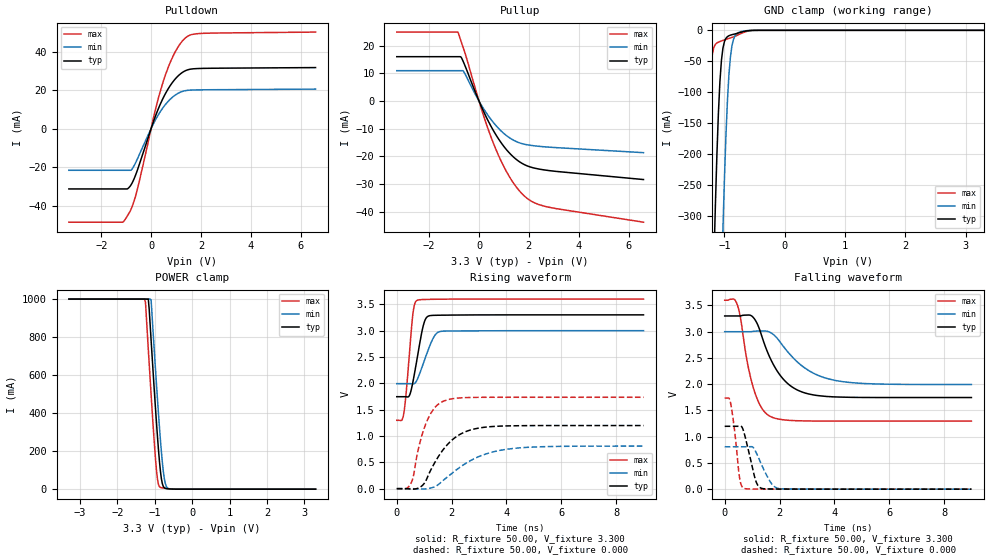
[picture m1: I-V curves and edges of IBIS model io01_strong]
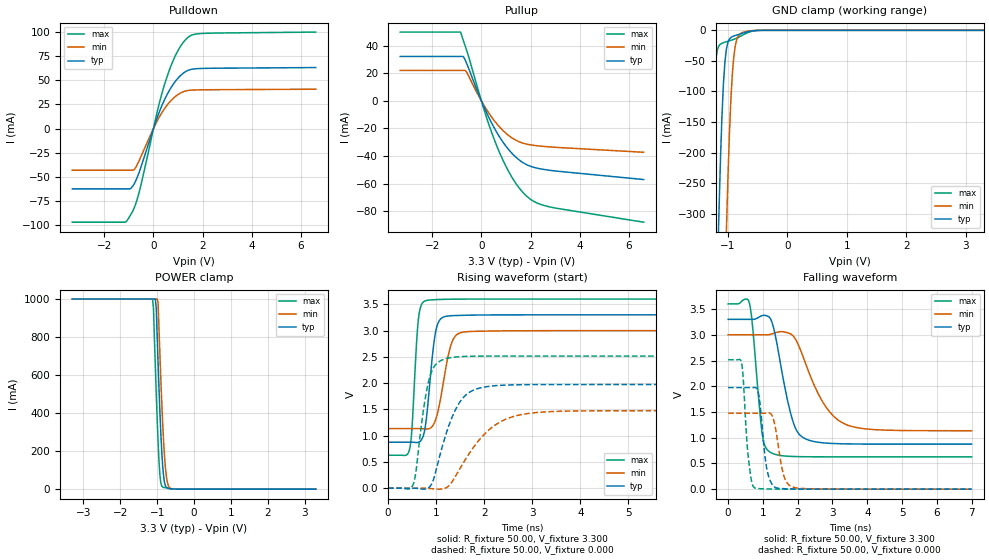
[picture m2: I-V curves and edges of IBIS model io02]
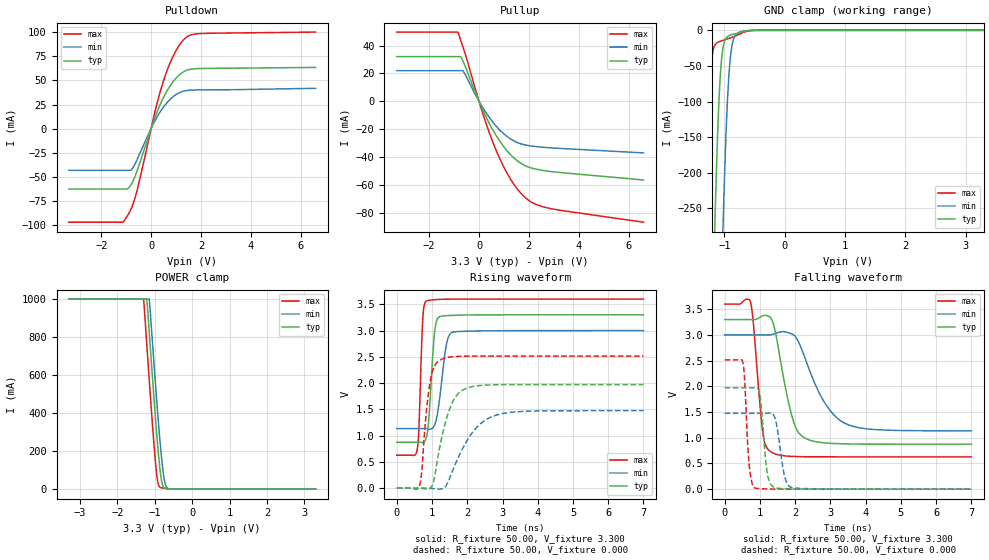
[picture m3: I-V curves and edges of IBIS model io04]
[IBIS Ver]   3.2
[File name]   rx63n_176lqfp.ibs
[File Rev]   1.00
[Date]   May 21, 2013
[Source]   From silicon level SPICE model at
   Renesas Electronics Corporation
[Notes]
|   Renesas Microcomputer RX631/RX63N Group
|   RX631/RX63N 176pin LQFP
|   VCCQ : 3.30V
|(1) This IBIS file checked the format with ibischk5.
|   Format Error and Warning are 0.
|(2) Temperature described Tj.
|   Tj[deg]
|   Typical   45.0
|   Minimum   105.0
|   Maximum   -40.0
|(3) History
|   Rev 0.50  2012.09.10
|   New creation by Renesas Electronics Corporation
|   Rev 1.00  2013.05.21
|   Only change of revision number.
|   by Renesas Electronics Corporation
[Disclaimer]
   This information is for modeling purposes only,
   and is not guaranteed.
[Copyright]   Copyright 2012, Renesas Electronics Corporation ,
   All Rights Reserved
[Component]   rx63n_176lqfp
[Manufacturer]  Renesas Electronics Corporation
[Package]
|   typ   min   max
R_pkg   254m   226m   289m
L_pkg   4.5nH   3.8nH   5.1nH
C_pkg   1.0pF   0.8pF   1.2pF
[Pin] signal_name   model_name
1   AVSS0   GND
2   P05   io02
3   VREFH   POWER
4   P03   io02
5   VREFL   GND
6   P02   io01
7   P01   io01
8   P00   io01
9   PF5   io04
10   EMLE   input06
11   PJ5   io04
12   VSS   GND
13   PJ3   io04
14   VCL   POWER
15   VBATT   POWER
16   NC   NC
17   PF4   io04
18   MD   io04
19   XCIN   NC
20   XCOUT   NC
21   RES#   input02
22   P37   io05
23   VSS   GND
24   P36   io03
25   VCC   POWER
26   P35   input01
27   P34   io04
28   P33   io06
29   P32   io21
30   PF3   io04
31   PF2   io04
32   P31   io21
33   P30   io21
34   PF1   io04
35   PF0   io04
36   P27   io07
37   P26   io07
38   P25   io04
39   VCC   POWER
40   P24   io04
41   VSS   GND
42   P23   io04
43   P22   io04
44   P21   io16
45   P20   io16
46   P17   io15
47   P87   io04
48   P16   io15
49   P86   io04
50   P15   io06
51   P14   io06
52   P85   io04
53   P13   io18
54   P12   io18
55   P11   io04
56   P10   io04
57   VCC_USB   POWER
58   USB0_DM   io09
59   USB0_DP   io09
60   VSS_USB   GND
61   P57   io07
62   P56   io07
63   USB1_DM   io09
64   USB1_DP   io09
65   VCC_USB   POWER
66   P55   io07
67   P54   io07
68   P53   io04
69   P84   io04
70   P52   io07
71   P51   io07
72   P50   io07
73   VSS   GND
74   P83   io04
75   VCC   POWER
76   PC7   io07
77   PC6   io07
78   PC5   io07
79   P82   io04
80   P81   io04
81   P80   io04
82   PC4   io07
83   PC3   io08
84   P77   io04
85   P76   io04
86   PC2   io08
87   P75   io04
88   P74   io04
89   PC1   io17
90   VCC   POWER
91   PC0   io17
92   VSS   GND
93   P73   io04
94   PB7   io07
95   PB6   io07
96   PB5   io07
97   PB4   io07
98   PB3   io07
99   PB2   io07
100   PB1   io07
101   P72   io04
102   P71   io04
103   VCC   POWER
104   PB0   io07
105   VSS   GND
106   PA7   io07
107   PA6   io07
108   PA5   io07
109   PA4   io07
110   PA3   io07
111   PG7   io07
112   PA2   io07
113   PG6   io07
114   PA1   io07
115   VCC   POWER
116   PG5   io04
117   VSS   GND
118   PA0   io07
119   PG4   io07
120   P67   io06
121   PG3   io07
122   P66   io04
123   PG2   io07
124   P65   io04
125   PE7   io01
126   PE6   io01
127   VCC   POWER
128   P70   io04
129   VSS   GND
130   PE5   io01
131   PE4   io01
132   PE3   io01
133   PE2   io01
134   PE1   io01
135   PE0   io01
136   P64   io04
137   P63   io04
138   P62   io04
139   P61   io04
140   VSS   GND
141   P60   io04
142   VCC   POWER
143   PD7   io01
144   PG1   io07
145   PD6   io01
146   PG0   io07
147   PD5   io01
148   PD4   io01
149   P97   io07
150   PD3   io01
151   VSS   GND
152   P96   io07
153   VCC   POWER
154   PD2   io01
155   P95   io07
156   PD1   io01
157   P94   io07
158   PD0   io01
159   P93   io01
160   P92   io01
161   P91   io01
162   VSS   GND
163   P90   io01
164   VCC   POWER
165   P47   io14
166   P46   io14
167   P45   io14
168   P44   io14
169   P43   io14
170   P42   io14
171   P41   io14
172   VREFL0   GND
173   P40   io14
174   VREFH0   POWER
175   AVCC0   POWER
176   P07   io06
[Diff Pin]   inv_pin   vdiff   tdelay_typ   tdelay_min   tdelay_max
58   59   0.000V   0.000s   NA   NA
63   64   0.000V   0.000s   NA   NA
[Model Selector]   io01
io01_strong   driver strength strong
io01_weak   driver strength weak
[Model Selector]   io07
io07_strong   driver strength strong
io07_weak   driver strength weak
[Model Selector]   io08
io08_strong   driver strength strong
io08_weak   driver strength weak
[Model Selector]   io15
io15a   driver strength strong
io15b   I2C buffer 1
[Model Selector]   io16
io16a   driver strength strong
io16b   I2C buffer 2
[Model Selector]   io17
io17a_strong   driver strength strong
io17a_weak   driver strength weak
io17b   I2C buffer 3
[Model Selector]   io18
io18a   driver strength strong
io18b   I2C buffer 4
| Models and submodels in the file (26): io01_strong (I/O), io01_weak (I/O), io02 (I/O), io03 (I/O), io04 (I/O), io05 (I/O), io06 (I/O), io07_strong (I/O), io07_weak (I/O), io08_strong (I/O), io08_weak (I/O), io09 (I/O), io14 (I/O), io15a (I/O), io15b (I/O_open_drain), io16a (I/O), io16b (I/O_open_drain), io17a_strong (I/O), io17a_weak (I/O), io17b (I/O_open_drain), io18a (I/O), io18b (I/O_open_drain), io21 (I/O), input01 (Input), input02 (Input), input06 (Input)
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[Model]   io01_strong
Model_type   I/O
Polarity   Non-Inverting
Enable   Active-High
Vinl  =   0.660V
Vinh  =   2.640V
Vmeas =   1.650V
Cref  =   30.00pF
| variable   typ   min   max
C_comp   5.910pF   5.910pF   5.910pF
| variable   typ   min   max
[Temperature Range]   45.000   105.000   -40.000
| variable   typ   min   max
[Voltage Range]   3.300V   3.000V   3.600V
| variable   typ   min   max
[Pullup Reference]   3.300V   3.000V   3.600V
| variable   typ   min   max
[Pulldown Reference]   0.000V   0.000V   0.000V
| variable   typ   min   max
[POWER Clamp Reference] 3.300V   3.000V   3.600V
| variable   typ   min   max
[GND Clamp Reference]   0.000V   0.000V   0.000V
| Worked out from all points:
|   slope of the pulldown table from 0 to 0.495 V, typ, clamps not added: 30.7 ohm
|   slope of the pullup table from 0 to 0.495 V, typ, clamps not added: 52.9 ohm
|   GND clamp passes 1 mA (typ) near -0.63 V on its own axis
|   POWER clamp passes 1 mA (typ) near -0.58 V on its own axis
|   rising waveform, R_fixture 50.00, V_fixture 3.300: 20-80 % time 321ps typ, 432ps min, 222ps max; typ from 1.75 V to 3.3 V
|   rising waveform, R_fixture 50.00, V_fixture 0.000: 20-80 % time 961ps typ, 1.48ns min, 553ps max; typ from 0 V to 1.2 V
|   falling waveform, R_fixture 50.00, V_fixture 3.300: 20-80 % time 902ps typ, 1.27ns min, 542ps max; typ from 3.3 V to 1.75 V
|   falling waveform, R_fixture 50.00, V_fixture 0.000: 20-80 % time 324ps typ, 446ps min, 218ps max; typ from 1.2 V to 0 V
[Pulldown]
| io01_strong Pulldown rx631_rx63n
| Thu Mar 22 17:15:49 2012
| voltage   I(typ)   I(min)   I(max)
-3.3V     -31.31mA   -21.63mA   -48.57mA
-1.15V    -31.31mA   -21.63mA   -48.57mA
-1.025V   -31.31mA   -21.63mA   -46.81mA
-800mV    -29.1mA    -21.49mA   -41.71mA
-600mV    -23.34mA   -17.13mA   -33.95mA
175mV     6.49mA     4.538mA    9.911mA
525mV     16.92mA    11.68mA    25.93mA
950mV     25.49mA    17.23mA    39.38mA
1.4V      30.18mA    19.75mA    47.31mA
1.7V      31.04mA    20.05mA    49.02mA
2.1V      31.26mA    20.14mA    49.45mA
6.6V      31.67mA    20.5mA     50.09mA
[Pullup]
| io01_strong Pullup rx631_rx63n
| Thu Mar 22 17:15:49 2012
| voltage   I(typ)   I(min)   I(max)
-3.3V     16.04mA    10.98mA    24.94mA
-850mV    16.04mA    10.98mA    24.94mA
-725mV    15.94mA    10.98mA    21.66mA
-625mV    14.1mA     10.75mA    19.05mA
175mV     -3.59mA    -2.649mA   -5.083mA
700mV     -12.53mA   -9.072mA   -17.96mA
1V        -16.45mA   -11.75mA   -23.79mA
1.325V    -19.76mA   -13.87mA   -28.89mA
1.95V     -23.51mA   -15.85mA   -35.33mA
2.3V      -24.41mA   -16.28mA   -37.1mA
2.9V      -25.25mA   -16.74mA   -38.59mA
6.6V      -28.4mA    -18.67mA   -43.82mA
[GND Clamp]
| io01_strong GNDClamp rx631_rx63n
| Thu Mar 22 17:15:49 2012
| voltage   I(typ)   I(min)   I(max)
-3.3V     -1A        -1A        -1A
-1.325V   -1A        -1A        -369.2mA
-1.3V     -928.6mA   -1A        -269.7mA
-1.25V    -694.8mA   -1A        -112.6mA
-1.175V   -376mA     -953.3mA   -27.44mA
-1.15V    -283.8mA   -837.7mA   -22.69mA
-1.075V   -83.42mA   -512.2mA   -18.16mA
-1.025V   -28.94mA   -323mA     -16.39mA
-925mV    -8.707mA   -71.38mA   -13.1mA
-850mV    -6.468mA   -14.65mA   -10.64mA
-675mV    -1.81mA    -1.082mA   -3.186mA
3.3V      0A         0A         0A
[POWER Clamp]
| io01_strong PWRClamp rx631_rx63n
| Thu Mar 22 17:15:49 2012
| voltage   I(typ)   I(min)   I(max)
-3.3V     1A         1A         1A
-1.275V   1A         1A         1A
-1.25V    1A         1A         982.1mA
-1.175V   1A         1A         736.6mA
-1.1V     784.3mA    995.9mA    498mA
-1V       476.2mA    683.1mA    204.7mA
-950mV    332.1mA    533mA      87.52mA
-875mV    143.3mA    321.7mA    12.76mA
-825mV    55.42mA    197.2mA    7.873mA
-750mV    8.12mA     59.94mA    5.513mA
-625mV    1.619mA    2.607mA    2.132mA
3.3V      0A         0A         0A
[Ramp]
dV/dt_r   0.719/960.74p  0.485/1.48n   1.041/552.35p
dV/dt_f   0.933/901.13p  0.604/1.27n   1.382/541.71p
R_load = 50.00ohm
[Rising Waveform]
| io01_strong Rising-High rx631_rx63n
| Thu Mar 22 17:15:49 2012
R_fixture = 50.00
V_fixture = 3.300
V_fixture_min = 3.000
V_fixture_max = 3.600
C_fixture = 0.00pF
| Time   V(typ)   V(min)   V(max)
0s        1.746V     1.994V     1.297V
250ps     1.746V     1.994V     1.413V
450ps     1.759V     1.994V     2.489V
580ps     2.004V     1.989V     3.28V
645ps     2.183V     1.996V     3.491V
740ps     2.465V     2.064V     3.575V
1.045ns   3.216V     2.49V      3.592V
1.35ns    3.291V     2.878V     3.596V
1.585ns   3.293V     2.985V     3.598V
9ns       3.3V       3V         3.6V
[Rising Waveform]
| io01_strong Rising-Low rx631_rx63n
| Thu Mar 22 17:15:49 2012
R_fixture = 50.00
V_fixture = 0.000
C_fixture = 0.00pF
| Time   V(typ)   V(min)   V(max)
0s        0V         0V         0V
510ps     -7mV       0V         95mV
605ps     -9mV       -1mV       236mV
840ps     25mV       -7mV       868mV
1.075ns   164mV      -4mV       1.25V
1.385ns   494mV      37mV       1.537V
1.755ns   781mV      183mV      1.672V
2.55ns    1.09V      490mV      1.729V
3.975ns   1.191V     745mV      1.735V
9ns       1.198V     808mV      1.735V
[Falling Waveform]
| io01_strong Falling-High rx631_rx63n
| Thu Mar 22 17:15:49 2012
R_fixture = 50.00
V_fixture = 3.300
V_fixture_min = 3.000
V_fixture_max = 3.600
C_fixture = 0.00pF
| Time   V(typ)   V(min)   V(max)
0s        3.3V       3V         3.6V
445ps     3.3V       3V         3.533V
575ps     3.301V     3V         3.268V
825ps     3.317V     3V         2.418V
1.03ns    3.279V     3.006V     1.959V
1.325ns   2.961V     3.013V     1.567V
1.65ns    2.506V     2.99V      1.39V
2.46ns    1.947V     2.523V     1.308V
3.835ns   1.763V     2.095V     1.297V
9ns       1.746V     1.994V     1.297V
[Falling Waveform]
| io01_strong Falling-Low rx631_rx63n
| Thu Mar 22 17:15:49 2012
R_fixture = 50.00
V_fixture = 0.000
C_fixture = 0.00pF
| Time   V(typ)   V(min)   V(max)
0s        1.198V     808mV      1.735V
210ps     1.198V     808mV      1.65V
350ps     1.198V     808mV      1.163V
545ps     1.199V     808mV      210mV
710ps     1.068V     808mV      13mV
1.12ns    182mV      727mV      3mV
1.35ns    15mV       460mV      1mV
1.71ns    4mV        104mV      1mV
2.015ns   2mV        10mV       0V
9ns       0V         0V         0V
[Model]   io02
Model_type   I/O
Polarity   Non-Inverting
Enable   Active-High
Vinl  =   0.660V
Vinh  =   2.640V
Vmeas =   1.650V
Cref  =   30.00pF
| variable   typ   min   max
C_comp   4.810pF   4.810pF   4.810pF
| variable   typ   min   max
[Temperature Range]   45.000   105.000   -40.000
| variable   typ   min   max
[Voltage Range]   3.300V   3.000V   3.600V
| variable   typ   min   max
[Pullup Reference]   3.300V   3.000V   3.600V
| variable   typ   min   max
[Pulldown Reference]   0.000V   0.000V   0.000V
| variable   typ   min   max
[POWER Clamp Reference] 3.300V   3.000V   3.600V
| variable   typ   min   max
[GND Clamp Reference]   0.000V   0.000V   0.000V
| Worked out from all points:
|   slope of the pulldown table from 0 to 0.495 V, typ, clamps not added: 15.3 ohm
|   slope of the pullup table from 0 to 0.495 V, typ, clamps not added: 26.5 ohm
|   GND clamp passes 1 mA (typ) near -0.60 V on its own axis
|   POWER clamp passes 1 mA (typ) near -0.56 V on its own axis
|   rising waveform, R_fixture 50.00, V_fixture 3.300: 20-80 % time 160ps typ, 229ps min, 107ps max; typ from 0.875 V to 3.3 V
|   rising waveform, R_fixture 50.00, V_fixture 0.000: 20-80 % time 439ps typ, 750ps min, 233ps max; typ from 0 V to 1.97 V
|   falling waveform, R_fixture 50.00, V_fixture 3.300: 20-80 % time 438ps typ, 788ps min, 230ps max; typ from 3.3 V to 0.875 V
|   falling waveform, R_fixture 50.00, V_fixture 0.000: 20-80 % time 184ps typ, 224ps min, 154ps max; typ from 1.97 V to 0 V
[Pulldown]
| io02_strong Pulldown rx631_rx63n
| Thu Mar 22 17:15:49 2012
| voltage   I(typ)   I(min)   I(max)
-3.3V     -62.65mA   -43.27mA   -97.17mA
-1.15V    -62.65mA   -43.27mA   -97.17mA
-1.025V   -62.65mA   -43.27mA   -93.54mA
-800mV    -58.14mA   -42.96mA   -83.35mA
-600mV    -46.61mA   -34.21mA   -67.78mA
175mV     12.96mA    9.063mA    19.79mA
550mV     35.03mA    24.16mA    53.7mA
950mV     50.92mA    34.42mA    78.67mA
1.4V      60.32mA    39.47mA    94.54mA
1.7V      62.04mA    40.07mA    97.97mA
2.1V      62.48mA    40.25mA    98.84mA
6.6V      63.3mA     40.84mA    100.1mA
[Pullup]
| io02_strong Pullup rx631_rx63n
| Thu Mar 22 17:15:49 2012
| voltage   I(typ)   I(min)   I(max)
-3.3V     32.07mA    21.98mA    49.71mA
-850mV    32.07mA    21.98mA    49.71mA
-725mV    31.79mA    21.98mA    43.1mA
-625mV    28.07mA    21.44mA    37.9mA
150mV     -6.167mA   -4.559mA   -8.713mA
675mV     -24.26mA   -17.6mA    -34.7mA
975mV     -32.23mA   -23.07mA   -46.52mA
1.3V      -39mA      -27.43mA   -56.92mA
1.925V    -46.81mA   -31.61mA   -70.21mA
2.3V      -48.81mA   -32.55mA   -74.14mA
2.8V      -50.28mA   -33.35mA   -76.77mA
6.6V      -56.92mA   -37.21mA   -87.76mA
[GND Clamp]
| io02_strong GNDClamp rx631_rx63n
| Thu Mar 22 17:15:49 2012
| voltage   I(typ)   I(min)   I(max)
-3.3V     -1A        -1A        -1A
-1.325V   -1A        -1A        -406.6mA
-1.3V     -983.2mA   -1A        -299.4mA
-1.225V   -615mA     -1A        -75.45mA
-1.175V   -395.1mA   -992.5mA   -30.98mA
-1.15V    -297.6mA   -869.7mA   -25.1mA
-1.075V   -87.49mA   -526mA     -20.19mA
-1.025V   -30.91mA   -328.2mA   -18.56mA
-925mV    -10.2mA    -71.04mA   -15.59mA
-850mV    -7.712mA   -14.99mA   -12.74mA
-675mV    -2.503mA   -1.438mA   -4.223mA
3.3V      0A         0A         0A
[POWER Clamp]
| io02_strong PWRClamp rx631_rx63n
| Thu Mar 22 17:15:49 2012
| voltage   I(typ)   I(min)   I(max)
-3.3V     1A         1A         1A
-1.125V   1A         1A         1A
-1.1V     1A         1A         952.1mA
-1.05V    1A         1A         650.2mA
-1.025V   951.6mA    1A         507.1mA
-975mV    665.2mA    983.6mA    250.2mA
-925mV    406mA      705.8mA    73.52mA
-850mV    120.7mA    345.8mA    11.13mA
-800mV    34.79mA    171.7mA    8.224mA
-750mV    9.544mA    66.61mA    6.556mA
-625mV    2.042mA    3.124mA    2.737mA
3.3V      0A         0A         0A
[Ramp]
dV/dt_r   1.184/438.21p  0.886/749.00p  1.509/232.71p
dV/dt_f   1.455/438.02p  1.119/787.01p  1.783/229.46p
R_load = 50.00ohm
[Rising Waveform]
| io02_strong Rising-High rx631_rx63n
| Thu Mar 22 17:15:49 2012
R_fixture = 50.00
V_fixture = 3.300
V_fixture_min = 3.000
V_fixture_max = 3.600
C_fixture = 0.00pF
| Time   V(typ)   V(min)   V(max)
0s        875mV      1.135V     628mV
445ps     876mV      1.135V     734mV
495ps     875mV      1.135V     1.111V
625ps     873mV      1.135V     3.163V
760ps     1.097V     1.13V      3.561V
975ps     2.901V     1.27V      3.589V
1.16ns    3.261V     2.067V     3.595V
1.345ns   3.284V     2.816V     3.598V
1.575ns   3.291V     2.973V     3.599V
7ns       3.3V       3V         3.6V
[Rising Waveform]
| io02_strong Rising-Low rx631_rx63n
| Thu Mar 22 17:15:49 2012
R_fixture = 50.00
V_fixture = 0.000
C_fixture = 0.00pF
| Time   V(typ)   V(min)   V(max)
0s        0V         0V         0V
520ps     0V         0V         67mV
840ps     9mV        -4mV       2.022V
965ps     227mV      -13mV      2.324V
1.155ns   880mV      -9mV       2.452V
1.39ns    1.472V     210mV      2.496V
1.65ns    1.799V     608mV      2.51V
2.09ns    1.938V     1.104V     2.515V
2.6ns     1.967V     1.363V     2.515V
7ns       1.974V     1.476V     2.515V
[Falling Waveform]
| io02_strong Falling-High rx631_rx63n
| Thu Mar 22 17:15:49 2012
R_fixture = 50.00
V_fixture = 3.300
V_fixture_min = 3.000
V_fixture_max = 3.600
C_fixture = 0.00pF
| Time   V(typ)   V(min)   V(max)
0s        3.3V       3V         3.6V
610ps     3.3V       3V         3.618V
700ps     3.299V     3V         3.177V
985ps     3.373V     3V         1.049V
1.205ns   3.323V     3.007V     719mV
1.815ns   1.429V     3.009V     637mV
2.145ns   1.007V     2.591V     631mV
2.74ns    900mV      1.672V     629mV
3.33ns    881mV      1.274V     628mV
7ns       875mV      1.135V     628mV
[Falling Waveform]
| io02_strong Falling-Low rx631_rx63n
| Thu Mar 22 17:15:49 2012
R_fixture = 50.00
V_fixture = 0.000
C_fixture = 0.00pF
| Time   V(typ)   V(min)   V(max)
0s        1.974V     1.476V     2.515V
385ps     1.974V     1.476V     2.454V
570ps     1.974V     1.476V     683mV
755ps     1.978V     1.476V     29mV
890ps     1.793V     1.476V     10mV
1.125ns   352mV      1.48V      4mV
1.36ns    32mV       1.19V      2mV
1.61ns    9mV        242mV      1mV
1.88ns    4mV        36mV       0V
7ns       0V         0V         0V
[Model]   io04
Model_type   I/O
Polarity   Non-Inverting
Enable   Active-High
Vinl  =   0.660V
Vinh  =   2.640V
Vmeas =   1.650V
Cref  =   30.00pF
| variable   typ   min   max
C_comp   4.420pF   4.420pF   4.420pF
| variable   typ   min   max
[Temperature Range]   45.000   105.000   -40.000
| variable   typ   min   max
[Voltage Range]   3.300V   3.000V   3.600V
| variable   typ   min   max
[Pullup Reference]   3.300V   3.000V   3.600V
| variable   typ   min   max
[Pulldown Reference]   0.000V   0.000V   0.000V
| variable   typ   min   max
[POWER Clamp Reference] 3.300V   3.000V   3.600V
| variable   typ   min   max
[GND Clamp Reference]   0.000V   0.000V   0.000V
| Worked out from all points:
|   slope of the pulldown table from 0 to 0.495 V, typ, clamps not added: 15.4 ohm
|   slope of the pullup table from 0 to 0.495 V, typ, clamps not added: 26.5 ohm
|   GND clamp passes 1 mA (typ) near -0.64 V on its own axis
|   POWER clamp passes 1 mA (typ) near -0.59 V on its own axis
|   rising waveform, R_fixture 50.00, V_fixture 3.300: 20-80 % time 137ps typ, 205ps min, 88.9ps max; typ from 0.875 V to 3.3 V
|   rising waveform, R_fixture 50.00, V_fixture 0.000: 20-80 % time 423ps typ, 741ps min, 213ps max; typ from 0 V to 1.97 V
|   falling waveform, R_fixture 50.00, V_fixture 3.300: 20-80 % time 429ps typ, 779ps min, 219ps max; typ from 3.3 V to 0.875 V
|   falling waveform, R_fixture 50.00, V_fixture 0.000: 20-80 % time 149ps typ, 194ps min, 116ps max; typ from 1.97 V to 0 V
[Pulldown]
| io04_strong Pulldown rx631_rx63n
| Thu Mar 22 17:15:49 2012
| voltage   I(typ)   I(min)   I(max)
-3.3V     -62.62mA   -43.25mA   -97.14mA
-1.15V    -62.62mA   -43.25mA   -97.14mA
-1.025V   -62.62mA   -43.25mA   -93.52mA
-800mV    -58.13mA   -42.94mA   -83.32mA
-600mV    -46.6mA    -34.2mA    -67.76mA
175mV     12.96mA    9.062mA    19.78mA
550mV     35.03mA    24.16mA    53.68mA
950mV     50.91mA    34.42mA    78.65mA
1.4V      60.32mA    39.47mA    94.53mA
1.7V      62.04mA    40.07mA    97.97mA
2.1V      62.47mA    40.25mA    98.84mA
6.6V      63.56mA    41.89mA    100.3mA
[Pullup]
| io04_strong Pullup rx631_rx63n
| Thu Mar 22 17:15:49 2012
| voltage   I(typ)   I(min)   I(max)
-3.3V     32.04mA    21.95mA    49.68mA
-850mV    32.04mA    21.95mA    49.68mA
-725mV    31.77mA    21.95mA    43.08mA
-625mV    28.06mA    21.43mA    37.88mA
150mV     -6.165mA   -4.558mA   -8.71mA
675mV     -24.25mA   -17.59mA   -34.7mA
1V        -32.82mA   -23.46mA   -47.4mA
1.3V      -39mA      -27.43mA   -56.91mA
1.925V    -46.81mA   -31.61mA   -70.21mA
2.3V      -48.81mA   -32.55mA   -74.14mA
2.9V      -50.5mA    -33.47mA   -77.15mA
6.6V      -56.53mA   -37.08mA   -86.83mA
[GND Clamp]
| io04_strong GNDClamp rx631_rx63n
| Thu Mar 22 17:15:49 2012
| voltage   I(typ)   I(min)   I(max)
-3.3V     -1A        -1A        -1A
-1.325V   -916.4mA   -1A        -321.6mA
-1.225V   -508.3mA   -1A        -56.05mA
-1.175V   -327.1mA   -831.8mA   -23.6mA
-1.15V    -246.5mA   -730.6mA   -19.51mA
-1.075V   -71.99mA   -445.9mA   -15.62mA
-1.025V   -24.89mA   -280.5mA   -14.09mA
-975mV    -11.12mA   -147.9mA   -12.65mA
-925mV    -7.484mA   -61.53mA   -11.26mA
-850mV    -5.559mA   -12.59mA   -9.146mA
-675mV    -1.555mA   -930uA     -2.738mA
3.3V      0A         0A         0A
[POWER Clamp]
| io04_strong PWRClamp rx631_rx63n
| Thu Mar 22 17:15:49 2012
| voltage   I(typ)   I(min)   I(max)
-3.3V     1A         1A         1A
-1.3V     1A         1A         1A
-1.225V   1A         1A         787.8mA
-1.2V     968.8mA    1A         716.2mA
-1.15V    827mA      1A         574.7mA
-975mV    353.5mA    532.6mA    124.6mA
-925mV    232.2mA    403.9mA    41.33mA
-875mV    126.2mA    282.6mA    11.35mA
-825mV    48.99mA    173.5mA    7.014mA
-750mV    7.221mA    53mA       4.912mA
-625mV    1.442mA    2.321mA    1.9mA
3.3V      0A         0A         0A
[Ramp]
dV/dt_r   1.184/423.57p  0.886/740.07p  1.509/212.85p
dV/dt_f   1.455/428.81p  1.119/778.62p  1.783/218.73p
R_load = 50.00ohm
[Rising Waveform]
| io04_strong Rising-High rx631_rx63n
| Thu Mar 22 17:15:49 2012
R_fixture = 50.00
V_fixture = 3.300
V_fixture_min = 3.000
V_fixture_max = 3.600
C_fixture = 0.00pF
| Time   V(typ)   V(min)   V(max)
0s        875mV      1.135V     628mV
575ps     876mV      1.135V     720mV
625ps     875mV      1.135V     1.101V
740ps     871mV      1.136V     3.247V
840ps     969mV      1.134V     3.562V
1.075ns   2.982V     1.207V     3.588V
1.205ns   3.261V     1.649V     3.593V
1.4ns     3.283V     2.704V     3.597V
1.57ns    3.289V     2.964V     3.599V
7ns       3.3V       3V         3.6V
[Rising Waveform]
| io04_strong Rising-Low rx631_rx63n
| Thu Mar 22 17:15:49 2012
R_fixture = 50.00
V_fixture = 0.000
C_fixture = 0.00pF
| Time   V(typ)   V(min)   V(max)
0s        0V         0V         0V
655ps     0V         0V         70mV
835ps     -17mV      0V         1.423V
945ps     1mV        -2mV       2.018V
1.06ns    173mV      -9mV       2.308V
1.245ns   869mV      -16mV      2.444V
1.705ns   1.772V     526mV      2.508V
2.195ns   1.94V      1.102V     2.514V
2.685ns   1.967V     1.358V     2.515V
7ns       1.973V     1.476V     2.515V
[Falling Waveform]
| io04_strong Falling-High rx631_rx63n
| Thu Mar 22 17:15:49 2012
R_fixture = 50.00
V_fixture = 3.300
V_fixture_min = 3.000
V_fixture_max = 3.600
C_fixture = 0.00pF
| Time   V(typ)   V(min)   V(max)
0s        3.3V       3V         3.6V
730ps     3.3V       3V         3.645V
810ps     3.299V     3V         3.25V
1.09ns    3.374V     3V         1.055V
1.325ns   3.313V     3.004V     720mV
1.91ns    1.416V     3.019V     637mV
2.245ns   1.005V     2.613V     631mV
2.85ns    899mV      1.667V     629mV
3.43ns    881mV      1.275V     628mV
7ns       875mV      1.135V     628mV
[Falling Waveform]
| io04_strong Falling-Low rx631_rx63n
| Thu Mar 22 17:15:49 2012
R_fixture = 50.00
V_fixture = 0.000
C_fixture = 0.00pF
| Time   V(typ)   V(min)   V(max)
0s        1.973V     1.476V     2.515V
515ps     1.973V     1.476V     2.467V
695ps     1.973V     1.476V     474mV
845ps     1.975V     1.476V     28mV
1ns       1.82V      1.476V     10mV
1.225ns   253mV      1.478V     4mV
1.415ns   31mV       1.405V     2mV
1.69ns    9mV        278mV      1mV
1.9ns     5mV        31mV       0V
7ns       0V         0V         0V
